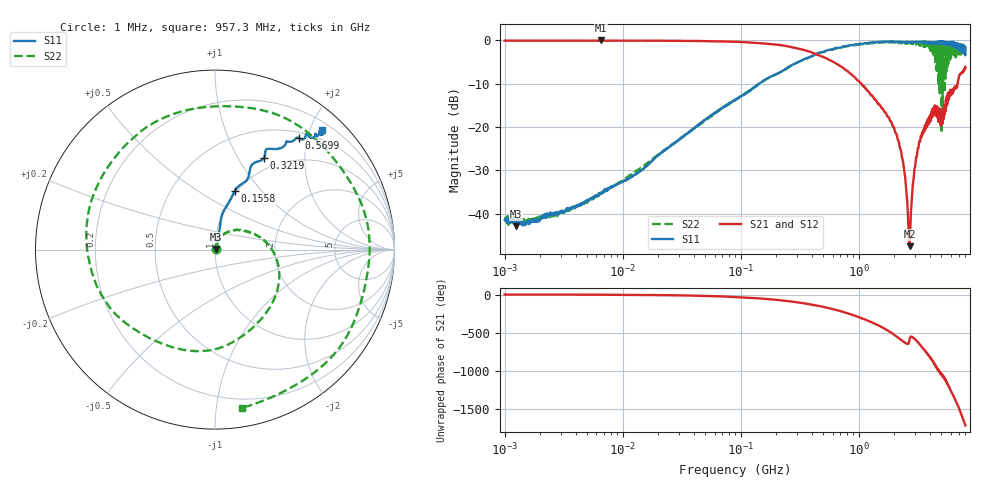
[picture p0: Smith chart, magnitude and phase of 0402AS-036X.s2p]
!s-Parameter Generated by FASTRON Sdn. Bhd.
!FASTRON P/N : 0402AS-036X
!Keysight Technologies: E5071C_MY46733604_B.14.02
!Date: Mon Dec 01 10:46:01 2025
!Version  :Rev00  Mon Dec 01 10:46:01 2025
!Data & Calibration Information:
!Freq  S11:SOLT2(ON)  S21:SOLT2(ON)  S12:SOLT2(ON)  S22:SOLT2(ON)
!PortZ  Port1:50+j0  Port2:50+j0
!When reading reference impedance value at option line is always used.
! Remarks : This data is being provided solely for informational purposes.
# Hz S dB R 50
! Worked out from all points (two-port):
!   1601 points, 1 MHz to 8 GHz, reference 50 ohm
!   highest |S21| = -0.03 dB at 6.532 MHz (marker M1); lowest = -47.5 dB at 2.692 GHz (marker M2)
!   |S21| within 3 dB of the highest: start of sweep to 420 MHz
!   lowest |S11| = -42.9 dB at 1.251 MHz (marker M3), VSWR 1.01, Z = 50.6 + j0.315 ohm
!   |S11| at or under -10 dB: start of sweep to 142.7 MHz
!   |S22| runs from -42.6 to -0.2 dB; largest |S21 - S12| = 0.019
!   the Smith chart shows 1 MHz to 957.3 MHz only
!   S11 on the Smith chart (normalised r, x): 1 MHz: 1.02, +0.01; 155.8 MHz: 0.98, +0.72; 321.9 MHz: 0.84, +1.29; 569.9 MHz: 0.59, +1.85; 957.3 MHz: 0.32, +2.19
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1000000  -41.50 20.1  -0.08 -0.4  -0.07 -0.4  -41.70 18.5
1250831  -42.90 25.7  -0.08 -0.5  -0.07 -0.5  -41.90 15.5
4479405  -37.60 54.8  -0.08 -1.7  -0.07 -1.7  -37.80 54.7
6531720  -35.50 61.2  -0.03 -2.5  -0.05 -2.0  -35.40 60.8
2.00676e7  -26.50 73.9  -0.10 -7.3  -0.10 -7.3  -26.40 69.2
8.994653e7  -13.70 78.1  -0.34 -32.1  -0.33 -32.0  -13.80 29.7
1.557817e8  -9.31 71.4  -0.72 -54.6  -0.72 -54.5  -9.41 -6.2
3.219106e8  -4.76 61.9  -2.04 -108.0  -2.03 -108.0  -4.77 -102.0
4.006501e8  -3.70 59.1  -2.80 -133.0  -2.79 -133.0  -3.60 -147.0
5.698649e8  -2.18 53.1  -4.59 179.0  -4.57 179.0  -2.20 123.0
9.573479e8  -0.96 48.3  -8.99 75.1  -8.98 75.0  -0.98 -80.2
1.341815e9  -0.47 54.3  -13.40 -16.3  -13.40 -16.3  -0.59 89.1
1.542898e9  -0.37 60.0  -15.40 -61.3  -15.50 -61.4  -0.42 -6.9
1.7949e9  -0.29 66.4  -17.80 -119.0  -17.80 -119.0  -0.48 -129.0
2.061212e9  -0.43 72.1  -21.40 -180.0  -21.40 -180.0  -0.37 103.0
2.252141e9  -0.51 75.1  -25.10 136.0  -25.00 136.0  -0.39 8.3
2.692309e9  -0.37 86.3  -47.50 133.0  -47.50 130.0  -0.71 149.0
3.000426e9  -0.43 94.4  -29.10 134.0  -29.10 134.0  -0.47 2.5
3.365624e9  -0.37 103.0  -22.20 45.7  -22.20 45.4  -1.21 171.0
3.730463e9  -0.66 112.0  -19.00 -34.3  -19.00 -34.9  -1.23 8.3
4.115571e9  -0.76 121.0  -16.50 -120.0  -16.50 -121.0  -1.24 -169.0
8e9  -1.55 -111.0  -6.30 90.0  -6.32 89.6  -3.41 126.0
